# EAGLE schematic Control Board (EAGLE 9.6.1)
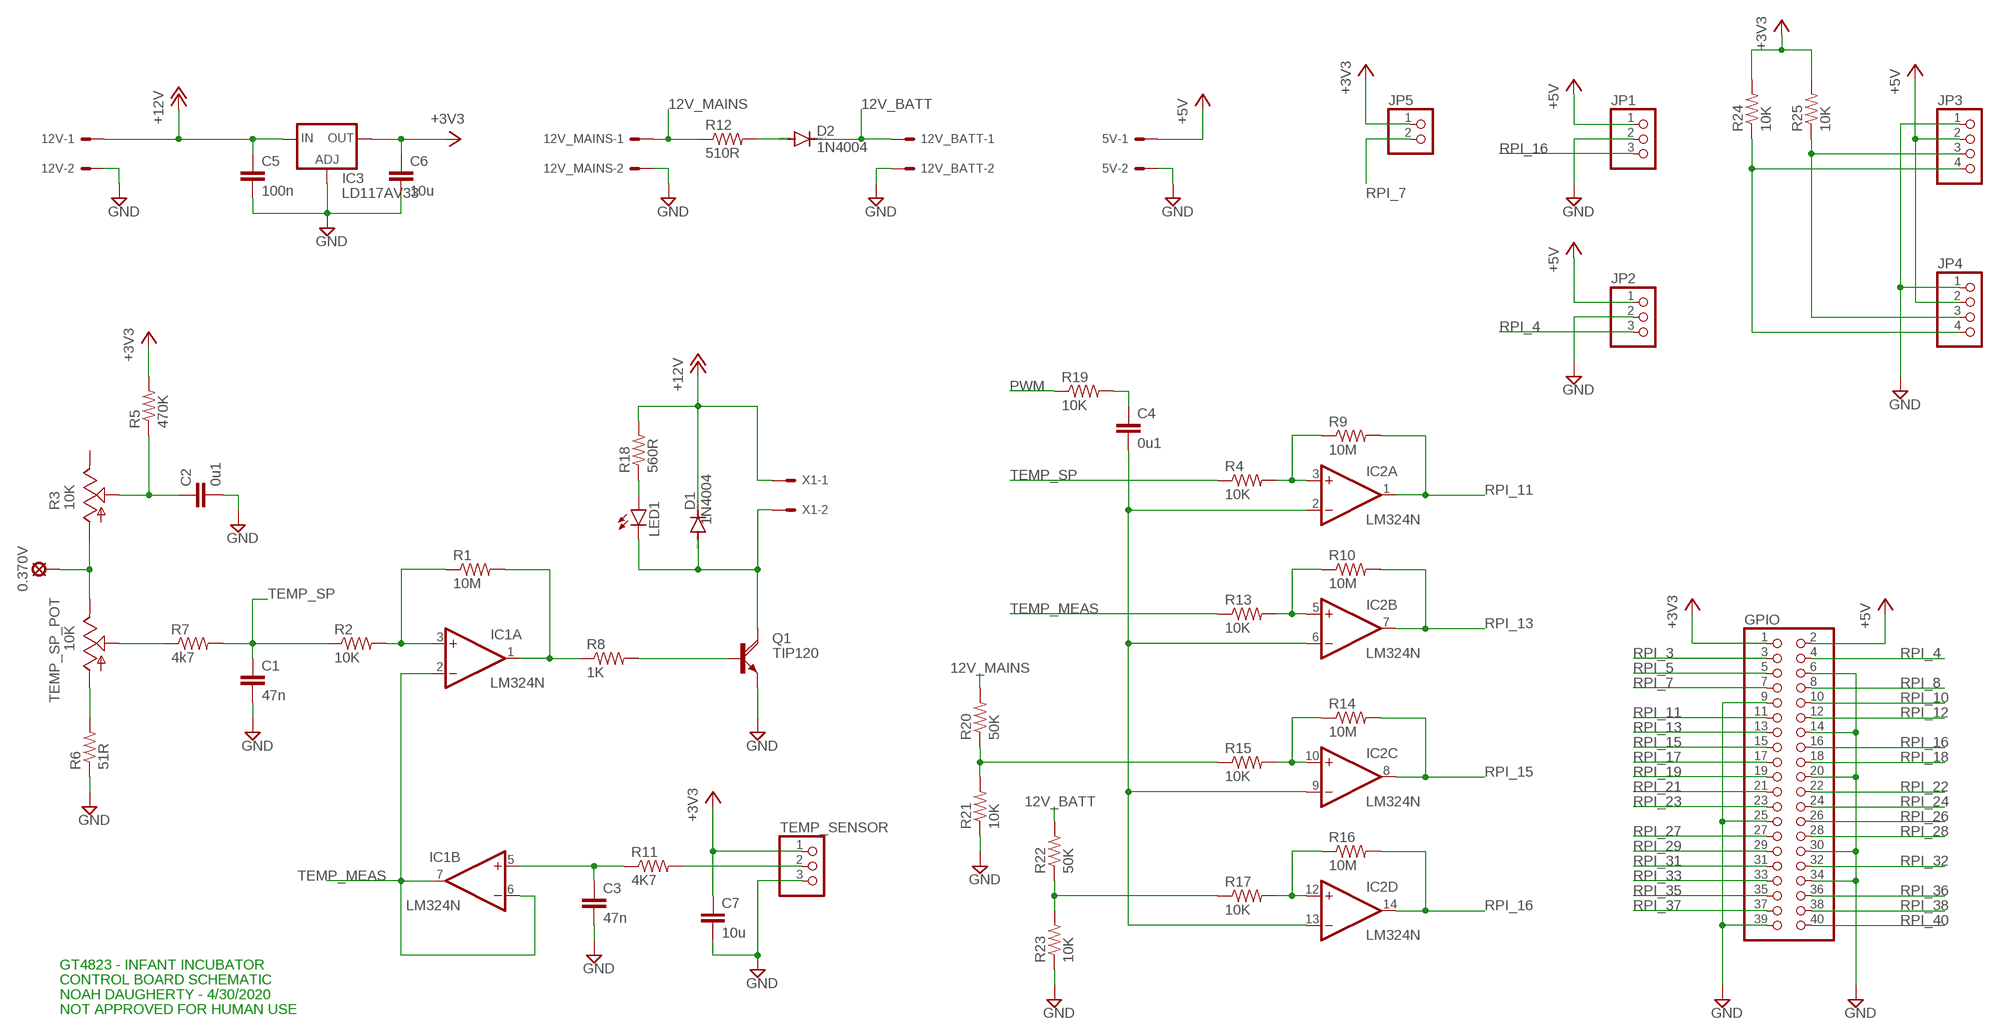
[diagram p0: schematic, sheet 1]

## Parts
0.370V  LSP10  [LSP10]
5V  KK-156-2  [KK-156-2]
12V  KK-156-2  [KK-156-2]
12V_BATT  KK-156-2  [KK-156-2]
12V_MAINS  KK-156-2  [KK-156-2]
C1  47n  C-EU050-025X075  [C050-025X075]
C2  0u1  C-EU050-025X075  [C050-025X075]
C3  47n  C-EU050-025X075  [C050-025X075]
C4  0u1  C-EU050-025X075  [C050-025X075]
C5  100n  C-EU050-025X075  [C050-025X075]
C6  10u  C-EU050-025X075  [C050-025X075]
C7  10u  C-EU050-025X075  [C050-025X075]
D1  1N4004  [DO41-10]
D2  1N4004  [DO41-10]
GPIO  PINHD-2X20  [2X20]
IC1  LM324N  [DIL14]
IC2  LM324N  [DIL14]
IC3  LD117AV33  [TO220L1]
JP1  PINHD-1X3  [1X03]
JP2  PINHD-1X3  [1X03]
JP3  PINHD-1X4  [1X04]
JP4  PINHD-1X4  [1X04]
JP5  PINHD-1X2  [1X02]
LED1  LED5MM  [LED5MM]
Q1  TIP120  [TO220AH]
R1  10M  R-US_0207/10  [0207/10]
R2  10K  R-US_0207/10  [0207/10]
R3  10K  TRIM_US-B25P  [B25P]
R4  10K  R-US_0207/10  [0207/10]
R5  470K  R-US_0207/10  [0207/10]
R6  51R  R-US_0207/10  [0207/10]
R7  4k7  R-US_0207/10  [0207/10]
R8  1K  R-US_0207/10  [0207/10]
R9  10M  R-US_0207/10  [0207/10]
R10  10M  R-US_0207/10  [0207/10]
R11  4K7  R-US_0207/10  [0207/10]
R12  510R  R-US_0207/10  [0207/10]
R13  10K  R-US_0207/10  [0207/10]
R14  10M  R-US_0207/10  [0207/10]
R15  10K  R-US_0207/10  [0207/10]
R16  10M  R-US_0207/10  [0207/10]
R17  10K  R-US_0207/10  [0207/10]
R18  560R  R-US_0207/10  [0207/10]
R19  10K  R-US_0207/10  [0207/10]
R20  50K  R-US_0207/10  [0207/10]
R21  10K  R-US_0207/10  [0207/10]
R22  50K  R-US_0207/10  [0207/10]
R23  10K  R-US_0207/10  [0207/10]
R24  10K  R-US_0207/10  [0207/10]
R25  10K  R-US_0207/10  [0207/10]
TEMP_SENSOR  PINHD-1X3  [1X03]
TEMP_SP_POT  10K  TRIM_US-B64Y  [B64Y]
X1  KK-156-2  [KK-156-2]

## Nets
12V_BATT: 12V_BATT.1 D2.C R22.2
12V_MAINS: 12V_MAINS.1 R12.1 R20.2
+3V3: C6.1 C7.1 GPIO.1 IC3.2(OUT) JP5.1 R5.2 R24.2 R25.2 TEMP_SENSOR.1
+5V: 5V.1 GPIO.2 JP1.1 JP2.1 JP3.2 JP4.2
+12V: 12V.1 C5.1 D1.C IC3.3(IN) R18.2 X1.1
GND: 5V.2 12V.2 12V_BATT.2 12V_MAINS.2 C1.2 C2.2 C3.2 C5.2 C6.2 C7.2 GPIO.6 GPIO.9 GPIO.14 GPIO.20 GPIO.25 GPIO.30 GPIO.34 GPIO.39 IC3.1(ADJ) JP1.2 JP2.2 JP3.1 JP4.1 Q1.E R6.1 R21.1 R23.1 TEMP_SENSOR.3
N$1: R15.1 R20.1 R21.2
N$2: 0.370V.MP R3.A TEMP_SP_POT.E
N$3: C2.1 R3.S R5.1
N$4: R6.2 TEMP_SP_POT.A
N$5: R7.1 TEMP_SP_POT.S
N$6: IC2.3(A:+IN) R4.2 R9.1
N$7: IC1.3(A:+IN) R1.1 R2.2
N$8: C3.1 IC1.5(B:+IN) R11.1
N$9: IC1.1(A:OUT) R1.2 R8.1
N$10: Q1.B R8.2
N$11: D1.A LED1.K(C) Q1.C X1.2
N$12: LED1.A R18.1
N$13: R17.1 R22.1 R23.2
N$15: D2.A R12.2
N$16: C4.1 R19.2
N$17: R11.2 TEMP_SENSOR.2
N$18: C4.2 IC2.2(A:-IN) IC2.6(B:-IN) IC2.9(C:-IN) IC2.13(D:-IN)
N$20: IC2.12(D:+IN) R16.1 R17.2
N$21: IC2.10(C:+IN) R14.1 R15.2
N$22: IC2.5(B:+IN) R10.1 R13.2
N$26: JP3.3 JP4.3 R25.1
N$27: JP3.4 JP4.4 R24.1
PWM: R19.1
RPI_3: GPIO.3
RPI_4: GPIO.4 JP2.3
RPI_5: GPIO.5
RPI_7: GPIO.7 JP5.2
RPI_8: GPIO.8
RPI_10: GPIO.10
RPI_11: GPIO.11 IC2.1(A:OUT) R9.2
RPI_12: GPIO.12
RPI_13: GPIO.13 IC2.7(B:OUT) R10.2
RPI_15: GPIO.15 IC2.8(C:OUT) R14.2
RPI_16: GPIO.16 IC2.14(D:OUT) JP1.3 R16.2
RPI_17: GPIO.17
RPI_18: GPIO.18
RPI_19: GPIO.19
RPI_21: GPIO.21
RPI_22: GPIO.22
RPI_23: GPIO.23
RPI_24: GPIO.24
RPI_26: GPIO.26
RPI_27: GPIO.27
RPI_28: GPIO.28
RPI_29: GPIO.29
RPI_31: GPIO.31
RPI_32: GPIO.32
RPI_33: GPIO.33
RPI_35: GPIO.35
RPI_36: GPIO.36
RPI_37: GPIO.37
RPI_38: GPIO.38
RPI_40: GPIO.40
TEMP_MEAS: IC1.2(A:-IN) IC1.6(B:-IN) IC1.7(B:OUT) R13.1
TEMP_SP: C1.1 R2.1 R4.1 R7.2
Unconnected: IC1.8(C:OUT) IC1.9(C:-IN) IC1.10(C:+IN) IC1.12(D:+IN) IC1.13(D:-IN) IC1.14(D:OUT) R3.E

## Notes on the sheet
- GT4823 - INFANT INCUBATOR
- CONTROL BOARD SCHEMATIC
- NOAH DAUGHERTY - 4/30/2020
- NOT APPROVED FOR HUMAN USE

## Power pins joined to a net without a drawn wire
V+: IC1.4(P:V+) IC2.4(P:V+)
V-: IC1.11(P:V-) IC2.11(P:V-)

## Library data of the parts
0.370V = solpad:LSP10: SOLDER PAD
5V 12V 12V_BATT 12V_MAINS X1 = con-molex:KK-156-2: KK 156 HEADER; MF: MOLEX; OC_FARNELL: unknown; OC_NEWARK: unknown
C1-C7 = rcl:C-EU: CAPACITOR, European symbol; SPICEPREFIX: C
D1 D2 = diode:1N4004: DIODE
GPIO = pinhead:PINHD-2X20: PIN HEADER
IC1 IC2 = linear:LM324: OP AMP
IC3 = v-reg:LD117A?*: Low drop fixed and adjustable positive voltage regulators 1 A Source: http://www.st.com/stonline/products/literature/ds/7194/ld1117axx.pdf
JP1 JP2 TEMP_SENSOR = pinhead:PINHD-1X3: PIN HEADER
JP3 JP4 = pinhead:PINHD-1X4: PIN HEADER
JP5 = pinhead:PINHD-1X2: PIN HEADER
LED1 = led:LED: LED
Q1 = transistor-power:TIP120: NPN DARLINGTON TRANSISTOR
R1 R2 R4-R25 = rcl:R-US_: RESISTOR, American symbol; SPICEPREFIX: R
R3 TEMP_SP_POT = pot:TRIM_US-: POTENTIOMETER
